PROGRAM MAIN
VAR
	iCounter : UDINT;
	fbAdsWrite : ADSWRITE;
	bWrite : BOOL := TRUE;
	fbTimer : TON;
	bOn : BOOL;
END_VAR

fbTimer(IN:=NOT bOn , PT:=T#1S , Q=> bOn  );

IF bOn THEN
	bWrite := TRUE;
	iCounter := iCounter +1;
ELSE
	bWrite := FALSE;
END_IF

fbAdsWrite(
	NETID:= '',
	PORT:= 27000,
	IDXGRP:= 16#20000,
	IDXOFFS:= 0,
	LEN:= SIZEOF(iCounter),
	SRCADDR:= ADR(iCounter),
	WRITE:=bWrite ,
	TMOUT:= T#50ms  );

END_PROGRAM
